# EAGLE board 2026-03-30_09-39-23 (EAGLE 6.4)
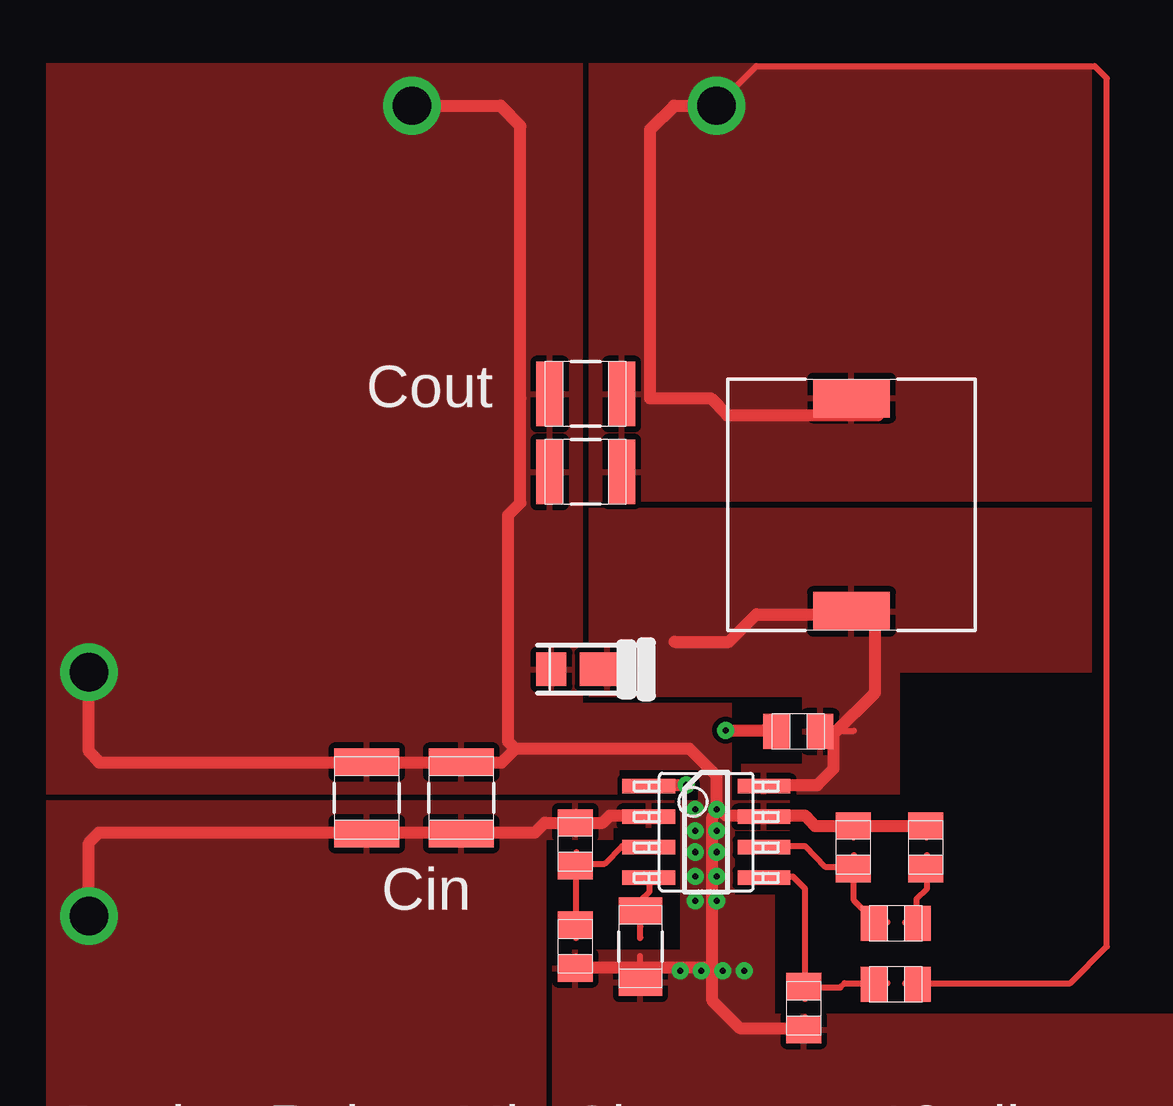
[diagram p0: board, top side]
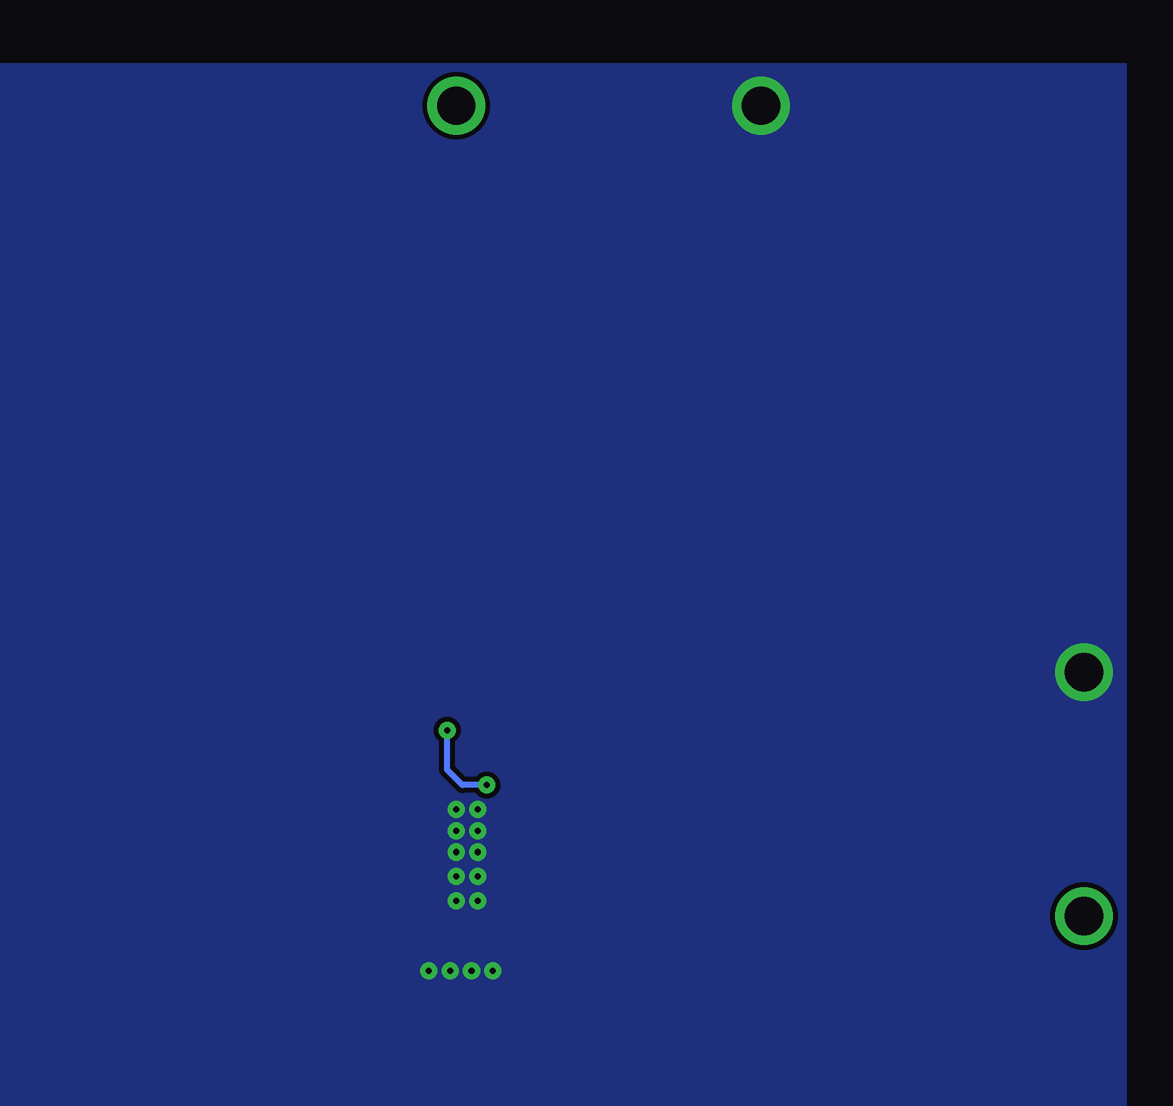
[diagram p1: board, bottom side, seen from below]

No outline drawn. Coordinates in mm, seen from the top.
Copper layers ((1*2)+(15*16)): TOP / INTERNAL1 / layer 15 / BOTTOM

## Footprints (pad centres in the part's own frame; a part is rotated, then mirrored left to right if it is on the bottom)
0805 = smd 1.118 x 1.448: 1 -0.902,0; 2 0.902,0
1210 = smd 1.118 x 2.692: 1 -1.499,0; 2 1.499,0
1210_280 = smd 1.118 x 2.692: 1 -1.499,0; 2 1.499,0
1206 = smd 1.118 x 1.803: 1 -1.499,0; 2 1.499,0
SOD-123HE = smd 2.3 x 1.4: 1 -0.9,0 | smd 1.25 x 1.4: 2 1.425,0
TP-1502 = drill 0.813 pad 1.651 round: 1 0,0
DR1040 = smd 1.6 x 3.2: 1 -4.445,0; 2 4.445,0
D0008A = smd 2.2 x 0.6: 1 -2.4,1.905; 2 -2.4,0.635; 3 -2.4,-0.635; 4 -2.4,-1.905; 5 2.4,-1.905; 6 2.4,-0.635; 7 2.4,0.635; 8 2.4,1.905

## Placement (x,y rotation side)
Cboot  [0805]  58.01,47.07 0 top
Ccomp  [0805]  63.32,42.24 90 top
Ccomp2  [0805]  60.3,42.24 90 top
Cin_1  [1210]  43.97,44.3 90 top
Cin_2  [1210]  40.03,44.3 90 top
Cout_1  [1210_280]  49.15,57.89 180 top
Cout_2  [1210_280]  49.15,61.14 180 top
Css  [1206]  51.44,38.1 270 top
D1  [SOD-123HE]  49.15,49.66 180 top
GND  [TP-1502]  28.45,49.48 0 top
GND1  [TP-1502]  41.88,73.13 0 top
L1  [DR1040]  60.22,56.52 270 top
Rcomp  [0805]  62.08,39.07 0 top
RenB  [0805]  48.72,38.1 270 top
RenT  [0805]  48.72,42.37 270 top
Rfbb  [0805]  58.24,35.53 270 top
Rfbt  [0805]  62.08,36.53 180 top
U1  [D0008A]  54.18,42.88 0 top
VIN  [TP-1502]  28.45,39.32 0 top
VOUT  [TP-1502]  54.58,73.13 0 top

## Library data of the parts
Cboot = ultra-librarian; RefDes: Cboot; Type: 08053C104KAT2A
Ccomp = ultra-librarian; RefDes: Ccomp; Type: CL21C102JBCNFNC
Ccomp2 = ultra-librarian; RefDes: Ccomp2; Type: CC0805JRNPO9BN100
Cin_1 Cin_2 Cout_1 Cout_2 = ultra-librarian
Css = ultra-librarian; RefDes: Css; Type: 12063A822JAT2A
D1 = ultra-librarian; RefDes: D1; Type: FSV360FP
GND = ultra-librarian; RefDes: GND; Type: TP-1502
GND1 = ultra-librarian; RefDes: GND1; Type: TP-1502
L1 = ultra-librarian; RefDes: L1; Type: DR1040-150-R
Rcomp = ultra-librarian; RefDes: Rcomp; Type: ERJ-6ENF4022V
RenB = ultra-librarian; RefDes: RenB; Type: CRCW080515K8FKEA
RenT = ultra-librarian; RefDes: RenT; Type: ERJ-6ENF1693V
Rfbb = ultra-librarian; RefDes: Rfbb; Type: ERJ-6ENF1961V
Rfbt = ultra-librarian; RefDes: Rfbt; Type: CRCW080510K2FKEA
U1 = ultra-librarian; RefDes: U1; Type: TPS54231DR
VIN = ultra-librarian; RefDes: VIN; Type: TP-1502
VOUT = ultra-librarian; RefDes: VOUT; Type: TP-1502

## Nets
0: Ccomp2.2 Ccomp.2 Cin_1.2 Cin_2.2 Cout_1.2 Cout_2.2 Css.2 D1.2 GND1.1 GND.1 RenB.2 Rfbb.2 U1.7
1: RenB.1 RenT.2 U1.3
2: Cboot.1 U1.1
3: Cin_1.1 Cin_2.1 RenT.1 U1.2 VIN.1
4: Ccomp.1 Rcomp.2
6: Ccomp2.1 Rcomp.1 U1.6
7: Rfbb.1 Rfbt.2 U1.5
8: Css.1 U1.4
9: Cout_1.1 Cout_2.1 L1.1 Rfbt.1 VOUT.1
10: Cboot.2 D1.1 L1.2 U1.8

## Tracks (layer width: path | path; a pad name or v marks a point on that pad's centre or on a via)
0  (via drill 0.25 pad 0.71, 1.6 pad 2.21)
  TOP 0.254: 58.28,34.21 58.28,35.15 | 60.31,42.65 60.31,43.59 | 63.36,42.65 63.36,43.59 | 51.42,36.75 51.42,37.69 | 48.76,36.75 48.76,37.69 | 63.37,43.13 | 63.88,43.13
  TOP 0.508: 63.37,43.13 60.33,43.13 58.7,43.13 58.29,43.56 56.62,43.56 54.99,43.56 54.74,43.81 54.43,43.51 54.43,37.24 | 48.77,37.24 54.43,37.24 | 54.43,37.24 54.43,35.84 55.58,34.7 58.29,34.7 | v41.91,73.15 45.59,73.15 46.43,72.29 46.43,60.96 46.43,56.59 45.92,56.08 45.92,50.8 45.92,46.63 46.23,46.35 | v28.45,49.53 28.45,46.23 28.88,45.77 42.29,45.77 45.64,45.77 46.23,46.35 | 46.23,46.35 53.47,46.35 54.61,45.21 v54.61,43.81
  other vias: 55.75,37.08 54.86,37.08 53.98,37.08 53.09,37.08 53.72,41.02 54.61,41.02 54.61,42.04 53.72,42.04 54.61,42.93 53.72,42.93 53.72,43.81 53.72,40.01 54.61,40.01
  pour TOP (rank 5): 26.67,44.45 50.55,44.45 50.55,45.47 53.85,45.47 53.85,44.2 53.09,44.2 53.09,37.97 47.75,37.97 47.75,26.67 74.93,26.67 74.93,35.31 57.02,35.31 57.02,40.26 55.37,40.26 55.37,42.93 57.66,42.93 57.66,44.2 55.24,44.2 55.24,48.26 49.02,48.26 49.02,74.93 26.67,74.93
  pour BOTTOM (rank 4): 74.93,26.67 74.93,74.93 26.67,74.93 26.67,26.67
1
  TOP 0.254: 48.77,38.48 48.77,38.94 48.77,41.55 | 48.77,41.55 48.77,42.04 | 48.77,41.55 49.94,41.55 50.67,42.29 51.82,42.29 | 48.76,38.46 48.76,39.4 | 48.76,41.07 48.76,42.01
2  (via drill 0.25 pad 0.71)
  TOP 0.254: 55.73,47.09 57.4,47.09
  TOP 0.508: 57.28,47.12 56.57,47.12 v54.99,47.12 | 51.82,44.83 v53.34,44.83
  BOTTOM 0.254: v53.34,44.83 54.36,44.83 54.99,45.47 54.99,46.99
3  (via drill 1.6 pad 2.21)
  TOP 0.254: 48.76,42.77 48.76,43.71
  TOP 0.508: v28.45,39.37 28.45,42.42 28.88,42.85 42.29,42.85 47.04,42.85 47.45,43.26 48.77,43.26 49.86,43.26 50.16,43.56 51.82,43.56
  pour TOP: 26.67,26.67 47.5,26.67 47.5,42.55 50.29,42.55 50.29,43.05 52.83,43.05 52.83,44.2 26.67,44.2
4
  TOP 0.254: 63.37,41.91 63.37,41.43 63.37,40.51 62.94,40.08 62.94,39.12 62.48,39.12 | 62.46,39.1 63.4,39.1 | 63.36,40.95 63.36,41.88
6
  TOP 0.254: 60.33,41.43 60.33,41.91 | 61.72,39.12 61.24,39.12 60.33,40.03 60.33,41.43 | 60.33,41.43 59.13,41.43 58.29,42.29 56.62,42.29 | 60.76,39.1 61.7,39.1 | 60.31,40.95 60.31,41.88
7
  TOP 0.254: 61.72,36.58 61.24,36.58 59.94,36.58 59.77,36.4 58.29,36.4 | 58.29,35.94 58.29,36.4 | 58.29,36.4 58.29,40.51 57.78,41.02 56.62,41.02 | 58.28,35.92 58.28,36.85 | 60.76,36.56 61.7,36.56
8
  TOP 0.254: 51.44,38.48 51.44,38.94 51.44,40.01 51.82,40.39 51.82,41.02 | 51.42,38.46 51.42,39.4
9  (via drill 1.6 pad 2.21)
  TOP 0.254: 62.48,36.58 62.94,36.58 | v54.61,73.15 56.26,74.8 70.36,74.8 70.87,74.3 70.87,38.1 69.34,36.58 63.45,36.58 | 62.46,36.56 63.4,36.56
  TOP 0.508: 61.34,60.25 55.04,60.25 54.36,60.96 51.84,60.96 51.84,72.16 52.83,73.15 v54.61,73.15
  pour TOP (rank 3): 70.23,74.93 49.28,74.93 49.28,56.64 70.23,56.64
10
  TOP 0.254: 58.65,47.09 60.33,47.09
  TOP 0.508: 52.86,50.8 55.12,50.8 56.26,51.94 61.01,51.94 61.21,51.74 61.21,48.69 59.49,46.99 59.49,45.52 58.8,44.83 56.62,44.83
  pour TOP (rank 2): 55.63,44.45 62.23,44.45 62.23,49.53 70.23,49.53 70.23,56.39 49.28,56.39 49.28,48.51 58.17,48.51 58.17,45.72 55.63,45.72

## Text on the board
ASSYNOTES: Cout | Cin | Design Rules: Min Clearance: 10mil | Min Track Width: 10mil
